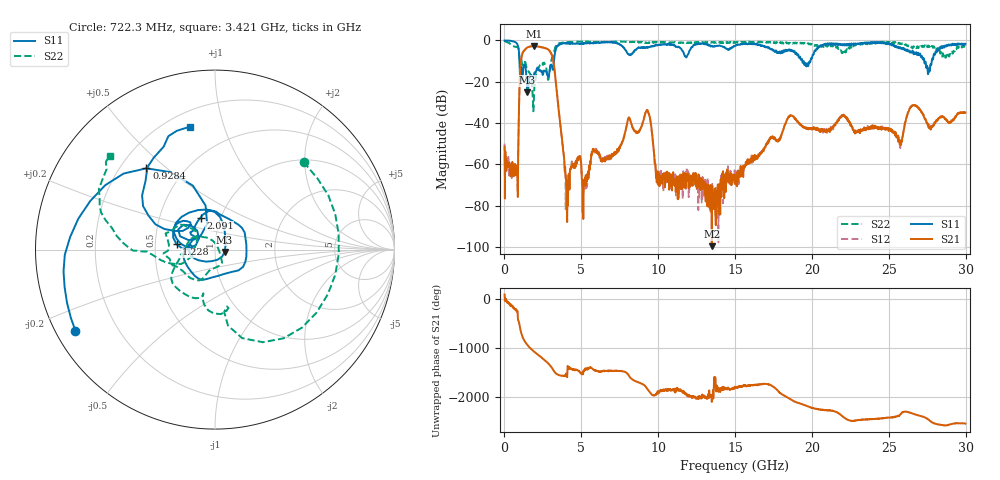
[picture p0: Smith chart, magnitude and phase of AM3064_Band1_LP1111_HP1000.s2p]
# Hz S DB R 50.0
!freq dBS11 angS11 dBS21 angS21 dBS12 angS12 dBS22 angS22
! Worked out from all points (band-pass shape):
!   1600 points, 10 MHz to 29.98 GHz, reference 50 ohm
!   highest |S21| = -2.78 dB at 1.922 GHz (marker M1); lowest = -99.7 dB at 13.49 GHz (marker M2)
!   |S21| within 3 dB of the highest: 1.203 GHz to 2.996 GHz (1.793 GHz wide, 85.4 % of centre)
!   lowest |S11| = -25.2 dB at 1.491 GHz (marker M3), VSWR 1.12, Z = 55.6 - j1.55 ohm
!   |S11| at or under -10 dB: 974.1 MHz to 3.219 GHz (2.245 GHz wide, 107 % of centre); 19.37 GHz to 19.9 GHz (532.3 MHz wide, 2.71 % of centre); 27.3 GHz to 27.8 GHz (495.9 MHz wide, 1.8 % of centre)
!   |S22| runs from -34.3 to -0.2 dB; largest |S21 - S12| = 0.013
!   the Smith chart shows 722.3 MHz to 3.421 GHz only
!   S11 on the Smith chart (normalised r, x): 722.3 MHz: 0.06, -0.27; 928.4 MHz: 0.31, +0.43; 1.228 GHz: 0.65, +0.04; 2.091 GHz: 0.80, +0.30; 3.421 GHz: 0.29, +0.77
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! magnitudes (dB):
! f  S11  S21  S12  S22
! 10 MHz  -0.1  -51.5  -50.0  -0.2
! 722.3 MHz  -0.9  -60.3  -62.5  -3.2
! 928.4 MHz  -4.5  -39.3  -39.3  -4.7
! 1.228 GHz  -13.3  -5.5  -5.4  -11.0
! 1.491 GHz  -25.2  -3.4  -3.4  -14.1
! 1.922 GHz  -16.6  -2.8  -2.8  -26.1
! 2.091 GHz  -14.2  -2.9  -2.9  -15.0
! 3.028 GHz  -11.8  -6.2  -6.1  -10.2
! 3.421 GHz  -3.1  -26.4  -26.3  -2.1
! 4.077 GHz  -1.4  -88.0  -81.8  -0.9
! 5.015 GHz  -1.5  -64.2  -63.3  -0.6
! 9.269 GHz  -3.2  -34.1  -33.6  -1.2
! 10 GHz  -2.2  -66.5  -70.0  -0.9
! 13.49 GHz  -2.6  -99.7  -75.3  -0.8
! 15 GHz  -2.7  -67.0  -63.8  -1.2
! 18.57 GHz  -5.1  -36.6  -36.4  -1.3
! 19.99 GHz  -8.8  -43.1  -42.9  -1.8
! 25 GHz  -1.4  -43.9  -42.8  -1.0
! 25.76 GHz  -3.9  -49.6  -49.2  -1.3
! 26.64 GHz  -6.5  -31.4  -31.4  -3.4
! 27.56 GHz  -16.3  -41.7  -41.7  -2.6
! 29.98 GHz  -1.7  -35.0  -35.1  -2.8
